|   TEXAS INSTRUMENTS INCORPORATED
|   Standard Linear and Logic
|   IBIS Model of SN74ALVCH162836
|   20-BIT Universal Bus Driver with 3-state outputs
|   56-pin DGG, DGV, or DL Package
[IBIS Ver]   2.1
[Comment char]  |_char
[File Name]   alvch162836.ibs
[File Rev]   2.0
[Date]   8/1/97
[Source]   File originated at Texas Instruments, Inc.
[Notes]   The following is an IBIS list for the ALVCH162836.
|   - This file may be incomplete or may not be fully compliant
|   with the IBIS specification. It will be replaced with a
|   version that is IBIS Revision 3.2 compliant and is complete
|   and accurate.  Please email all questions and comments to
|   sllibis@ti.com.
|   - All test data contained in this file are derived from
|   hspice(tm) simulations.
|   - File created by Ramzi Ammar, SLL Applications
[Disclaimer]
* Property of Texas Instruments Incorporated.  Unauthorized *
* reproduction and/or distribution is strictly prohibited. *
* This product is protected under copyright law. *
* Created 1997, (C) Copyright 1997, Texas Instruments Inc., *
* All Rights Reserved *
* UNLESS THERE IS A SIGNED, WRITTEN AGREEMENT TO THE *
* CONTRARY, TEXAS INSTRUMENTS ("TI") IS PROVIDING THE IBIS *
* MODELS "AS IS" AND WITHOUT ANY WARRANTY, EXPRESSED OR *
* IMPLIED.  TI assumes no liability for: *
* 1) the accuracy of the IBIS models provided to your *
* company; *
* 2) the proper functioning of these IBIS models in your *
* design or for any resulting applications; or *
* 3) infringement of patents, copyrights or intellectual *
* property rights resulting from your use of these *
* IBIS models. *
* TI provides IBIS Models as a service to our customers. *
* You and your company shall not distribute, sell or give *
* these models to anyone else without prior written *
* permission from TI. *
* TI reserves the right to make changes to our products or *
* to discontinue any semiconductor product or service *
* without notice, and advises our customers to obtain the *
* latest version of relevant information to verify, before *
* placing orders, that the information being relied on is *
* current. *
* Please be aware that your receipt and use of the IBIS *
* information provided shall serve as acceptance of these *
* terms and conditions.  If you do not accept these terms, *
* you should return or destroy the IBIS models and any *
* other accompanying information immediately. *
[Component]   ALVCH162836_DGG
[Manufacturer]  Texas Instruments, Inc.
[Package]
|   typ   min   max
R_pkg   0.035   0.029   0.046
L_pkg   3.072nH   2.572nH   4.265nH
C_pkg   0.518pF   0.393pF   0.677pF
[Pin]   signal_name   model_name   R_pin   L_pin   C_pin
1   OE_BAR   NC   0.039   4.225nH   0.65pF
2   Y1   OUT   0.037   3.732nH   0.657pF
3   Y2   OUT   0.044   3.552nH   0.639pF
4   GND   GND   0.029   3.383nH   0.621pF
5   Y3   OUT   0.029   3.239nH   0.621pF
6   Y4   OUT   0.03   3.06nH   0.574pF
7   VCC   POWER   0.033   2.95nH   0.512pF
8   Y5   OUT   0.033   2.809nH   0.469pF
9   Y6   OUT   0.032   2.695nH   0.443pF
10   Y7   OUT   0.034   2.666nH   0.43pF
11   GND   GND   0.035   2.619nH   0.407pF
12   Y8   OUT   0.037   2.618nH   0.4pF
13   Y9   OUT   0.037   2.634nH   0.402pF
14   Y10   OUT   0.039   2.655nH   0.405pF
15   Y11   OUT   0.038   2.599nH   0.401pF
16   Y12   OUT   0.037   2.603nH   0.399pF
17   Y13   OUT   0.038   2.638nH   0.402pF
18   GND   GND   0.037   2.702nH   0.413pF
19   Y14   OUT   0.036   2.75nH   0.436pF
20   Y15   OUT   0.034   2.76nH   0.447pF
21   Y16   OUT   0.033   2.839nH   0.472pF
22   VCC   POWER   0.032   2.965nH   0.516pF
23   Y17   OUT   0.029   3.007nH   0.587pF
24   Y18   OUT   0.029   3.222nH   0.633pF
25   GND   GND   0.029   3.382nH   0.621pF
26   Y19   OUT   0.042   3.536nH   0.639pF
27   Y20   OUT   0.039   3.8nH   0.677pF
28   NC   NC   0.039   4.265nH   0.66pF
29   LE_BAR   NC   0.038   4.224nH   0.651pF
30   A20   IN   0.037   3.742nH   0.663pF
31   A19   IN   0.046   3.598nH   0.64pF
32   GND   GND   0.032   3.41nH   0.617pF
33   A18   IN   0.03   3.26nH   0.626pF
34   A17   IN   0.03   3.083nH   0.586pF
35   VCC   POWER   0.031   2.943nH   0.513pF
36   A16   IN   0.033   2.889nH   0.473pF
37   A15   IN   0.034   2.812nH   0.449pF
38   A14   IN   0.035   2.742nH   0.433pF
39   GND   GND   0.036   2.678nH   0.407pF
40   A13   IN   0.036   2.614nH   0.394pF
41   A12   IN   0.039   2.65nH   0.396pF
42   A11   IN   0.038   2.572nH   0.395pF
43   A10   IN   0.038   2.614nH   0.399pF
44   A9   IN   0.037   2.64nH   0.396pF
45   A8   IN   0.037   2.615nH   0.393pF
46   GND   GND   0.036   2.642nH   0.404pF
47   A7   IN   0.036   2.707nH   0.43pF
48   A6   IN   0.034   2.733nH   0.443pF
49   A5   IN   0.034   2.825nH   0.467pF
50   VCC   POWER   0.033   2.945nH   0.513pF
51   A4   IN   0.031   3.03nH   0.584pF
52   A3   IN   0.031   3.279nH   0.634pF
53   GND   GND   0.031   3.393nH   0.618pF
54   A2   IN   0.042   3.507nH   0.634pF
55   A1   IN   0.039   3.781nH   0.666pF
56   CLK   NC   0.037   4.215nH   0.65pF
[Component]   ALVCH162836_DGV
[Manufacturer]  Texas Instruments, Inc.
[Package]
|   typ   min   max
R_pkg   0.056   0.025   0.1
L_pkg   2.961nH   1.897nH   4.848nH
C_pkg   0.397pF   0.244pF   0.659pF
[Pin]   signal_name   model_name   R_pin   L_pin   C_pin
1   OE_BAR   NC   0.1   4.848nH   0.659pF
2   Y1   OUT   0.096   4.436nH   0.65pF
3   Y2   OUT   0.095   4.138nH   0.568pF
4   GND   GND   0.098   3.897nH   0.495pF
5   Y3   OUT   0.082   3.448nH   0.443pF
6   Y4   OUT   0.068   3.096nH   0.392pF
7   VCC   POWER   0.056   2.728nH   0.384pF
8   Y5   OUT   0.027   2.483nH   0.36pF
9   Y6   OUT   0.027   2.397nH   0.309pF
10   Y7   OUT   0.028   2.304nH   0.302pF
11   GND   GND   0.029   2.179nH   0.28pF
12   Y8   OUT   0.03   2.045nH   0.268pF
13   Y9   OUT   0.032   2.003nH   0.259pF
14   Y10   OUT   0.033   1.951nH   0.249pF
15   Y11   OUT   0.033   1.963nH   0.25pF
16   Y12   OUT   0.032   2.008nH   0.259pF
17   Y13   OUT   0.03   2.034nH   0.267pF
18   GND   GND   0.03   2.141nH   0.276pF
19   Y14   OUT   0.029   2.33nH   0.302pF
20   Y15   OUT   0.028   2.402nH   0.308pF
21   Y16   OUT   0.027   2.459nH   0.354pF
22   VCC   POWER   0.054   2.694nH   0.377pF
23   Y17   OUT   0.064   2.958nH   0.381pF
24   Y18   OUT   0.08   3.384nH   0.438pF
25   GND   GND   0.096   3.829nH   0.488pF
26   Y19   OUT   0.097   4.096nH   0.562pF
27   Y20   OUT   0.093   4.354nH   0.643pF
28   NC   NC   0.096   4.753nH   0.641pF
29   LE_BAR   NC   0.094   4.721nH   0.64pF
30   A20   IN   0.089   4.276nH   0.633pF
31   A19   IN   0.089   4.015nH   0.555pF
32   GND   GND   0.096   3.852nH   0.488pF
33   A18   IN   0.079   3.379nH   0.438pF
34   A17   IN   0.065   2.984nH   0.384pF
35   VCC   POWER   0.054   2.682nH   0.375pF
36   A16   IN   0.026   2.451nH   0.353pF
37   A15   IN   0.026   2.334nH   0.302pF
38   A14   IN   0.028   2.289nH   0.297pF
39   GND   GND   0.027   2.104nH   0.272pF
40   A13   IN   0.029   2.009nH   0.263pF
41   A12   IN   0.031   1.955nH   0.254pF
42   A11   IN   0.031   1.902nH   0.245pF
43   A10   IN   0.031   1.897nH   0.244pF
44   A9   IN   0.03   1.955nH   0.254pF
45   A8   IN   0.029   2.024nH   0.265pF
46   GND   GND   0.028   2.133nH   0.275pF
47   A7   IN   0.028   2.305nH   0.299pF
48   A6   IN   0.027   2.376nH   0.305pF
49   A5   IN   0.025   2.47nH   0.359pF
50   VCC   POWER   0.056   2.72nH   0.383pF
51   A4   IN   0.064   2.983nH   0.387pF
52   A3   IN   0.081   3.408nH   0.441pF
53   GND   GND   0.095   3.872nH   0.492pF
54   A2   IN   0.098   4.142nH   0.564pF
55   A1   IN   0.096   4.428nH   0.64pF
56   CLK   NC   0.095   4.772nH   0.649pF
[Component]   ALVCH162836_DL
[Manufacturer]  Texas Instruments, Inc.
[Package]
|   typ   min   max
R_pkg   0.055   0.048   0.067
L_pkg   6.539nH   4.802nH   9.746nH
C_pkg   0.857pF   0.5pF   1.351pF
[Pin]   signal_name   model_name   R_pin   L_pin   C_pin
1   OE_BAR   NC   0.064   9.646nH   1.202pF
2   Y1   OUT   0.059   8.723nH   1.348pF
3   Y2   OUT   0.059   8.139nH   1.223pF
4   GND   GND   0.056   7.554nH   1.088pF
5   Y3   OUT   0.054   6.991nH   0.966pF
6   Y4   OUT   0.053   6.659nH   0.973pF
7   VCC   POWER   0.055   6.321nH   0.905pF
8   Y5   OUT   0.055   5.942nH   0.713pF
9   Y6   OUT   0.057   5.767nH   0.678pF
10   Y7   OUT   0.054   5.459nH   0.631pF
11   GND   GND   0.051   5.224nH   0.638pF
12   Y8   OUT   0.048   5.088nH   0.601pF
13   Y9   OUT   0.05   5.021nH   0.518pF
14   Y10   OUT   0.051   4.802nH   0.5pF
15   Y11   OUT   0.051   4.803nH   0.5pF
16   Y12   OUT   0.05   5.021nH   0.518pF
17   Y13   OUT   0.048   5.088nH   0.601pF
18   GND   GND   0.051   5.224nH   0.638pF
19   Y14   OUT   0.054   5.459nH   0.631pF
20   Y15   OUT   0.057   5.768nH   0.677pF
21   Y16   OUT   0.055   5.942nH   0.715pF
22   VCC   POWER   0.055   6.321nH   0.907pF
23   Y17   OUT   0.053   6.659nH   0.972pF
24   Y18   OUT   0.054   6.991nH   0.966pF
25   GND   GND   0.056   7.554nH   1.087pF
26   Y19   OUT   0.059   8.139nH   1.223pF
27   Y20   OUT   0.059   8.727nH   1.351pF
28   NC   NC   0.067   9.746nH   1.21pF
29   LE_BAR   NC   0.063   9.63nH   1.203pF
30   A20   IN   0.06   8.751nH   1.349pF
31   A19   IN   0.06   8.184nH   1.224pF
32   GND   GND   0.056   7.543nH   1.087pF
33   A18   IN   0.054   7.005nH   0.969pF
34   A17   IN   0.056   6.714nH   0.975pF
35   VCC   POWER   0.058   6.384nH   0.909pF
36   A16   IN   0.057   5.976nH   0.717pF
37   A15   IN   0.057   5.743nH   0.677pF
38   A14   IN   0.055   5.469nH   0.631pF
39   GND   GND   0.055   5.328nH   0.644pF
40   A13   IN   0.052   5.189nH   0.606pF
41   A12   IN   0.052   5.053nH   0.519pF
42   A11   IN   0.052   4.825nH   0.502pF
43   A10   IN   0.054   4.896nH   0.506pF
44   A9   IN   0.052   5.093nH   0.521pF
45   A8   IN   0.051   5.179nH   0.608pF
46   GND   GND   0.054   5.314nH   0.645pF
47   A7   IN   0.055   5.511nH   0.632pF
48   A6   IN   0.057   5.77nH   0.677pF
49   A5   IN   0.055   5.956nH   0.716pF
50   VCC   POWER   0.055   6.32nH   0.905pF
51   A4   IN   0.052   6.621nH   0.968pF
52   A3   IN   0.053   6.974nH   0.966pF
53   GND   GND   0.057   7.571nH   1.089pF
54   A2   IN   0.057   8.097nH   1.219pF
55   A1   IN   0.059   8.723nH   1.349pF
56   CLK   NC   0.061   9.56nH   1.199pF
| Models and submodels in the file (2): OUT (3-state), IN (Input)
